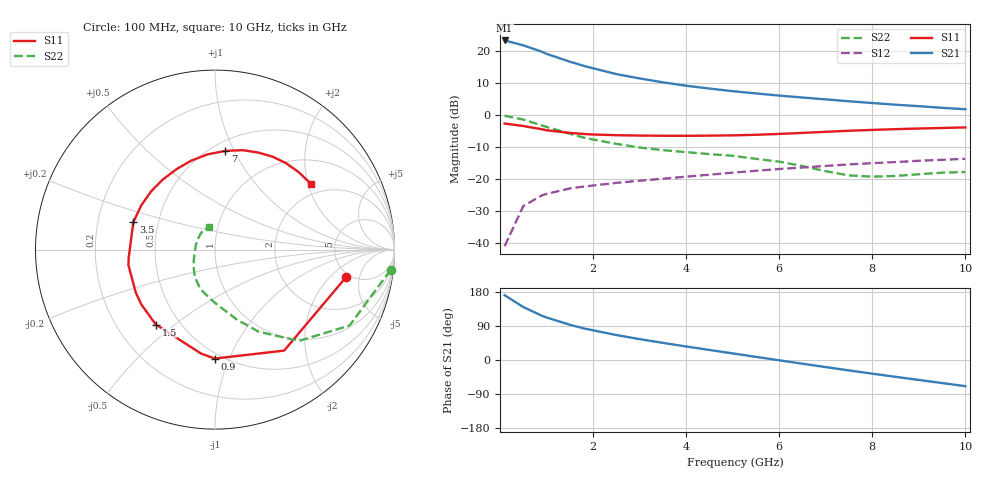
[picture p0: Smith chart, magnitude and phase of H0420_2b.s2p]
!HBFP-0420
!S-PARAMETERS at Vce=2V  Ic=5mA.  LAST UPDATED 05-29-98
# ghz s ma r 50
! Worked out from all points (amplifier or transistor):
!   23 points, 100 MHz to 10 GHz, reference 50 ohm
!   highest |S21| = 23.4 dB at 100 MHz (marker M1)
!   |S21| within 3 dB of that: start of sweep to 796.8 MHz
!   unconditionally stable (mu >= 1): 3.008 GHz to end of sweep
!   at 1 GHz: K = 0.39, MSG = 21.9 dB, |S12| = -24.6 dB
!   at 4.5 GHz: K = 1.20, MAG = 10.8 dB, |S12| = -18.6 dB
!   at 10 GHz: K = 1.24, MAG = 4.8 dB, |S12| = -13.6 dB
!   lowest NFmin = 1.00 dB at 900 MHz
!   S11 on the Smith chart (normalised r, x): 100 MHz: 4.59, -3.19; 900 MHz: 0.46, -0.89; 1.5 GHz: 0.37, -0.43; 3.5 GHz: 0.36, +0.14; 7 GHz: 0.58, +0.92; 10 GHz: 1.65, +2.09
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0.1  0.746 -11.9  14.85 171.0  0.009 84.8  0.985 -6.6
0.5  0.682 -55.6  12.47 139.8  0.038 63.6  0.861 -29.4
0.9  0.607 -90.1  9.909 116.8  0.056 49.3  0.696 -46.6
1  0.585 -97.5  9.181 112.2  0.059 46.9  0.661 -49.3
1.5  0.532 -128.3  6.918 93.1  0.072 37.2  0.516 -62.2
1.8  0.512 -143.1  5.952 83.4  0.077 33.2  0.45 -67.7
2  0.502 -151.6  5.453 78.4  0.08 31.2  0.419 -71.6
2.5  0.49 -169.8  4.422 65.8  0.088 26.9  0.359 -78.4
3  0.483 -174.6  3.786 55.2  0.095 23.4  0.314 -86.3
3.5  0.48 161.4  3.286 45.2  0.102 19.8  0.286 -92.5
4  0.479 149.2  2.908 35.7  0.11 16.3  0.266 -98.1
4.5  0.482 137.6  2.629 26.5  0.118 12.5  0.248 -104.1
5  0.487 126.5  2.389 17.4  0.127 8.1  0.233 -110.5
5.5  0.497 115.4  2.205 8.3  0.136 3.5  0.209 -117.9
6  0.513 105.0  2.04 -0.8  0.145 -1.5  0.189 -126.4
6.5  0.532 94.6  1.902 -9.8  0.153 -7.1  0.161 -137.1
7  0.553 84.0  1.778 -18.7  0.162 -12.6  0.134 -152.0
7.5  0.575 74.5  1.662 -27.5  0.171 -18.2  0.115 -171.2
8  0.592 66.0  1.559 -36.1  0.179 -24.0  0.11 167.1
8.5  0.609 58.2  1.469 -44.4  0.186 -29.8  0.113 147.2
9  0.623 50.7  1.393 -52.6  0.195 -35.4  0.12 130.6
10  0.648 34.5  1.248 -69.1  0.209 -48.0  0.13 103.9
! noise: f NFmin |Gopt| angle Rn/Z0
0.9  1  0.281  28.8  0.19
1.5  1.1  0.187  68.3  0.15
2  1.18  0.154  118.4  0.12
3  1.32  0.226  165.9  0.1
4  1.49  0.292  -162.3  0.1
5.5  1.75  0.375  -121  0.19
6.5  1.94  0.453  -98.1  0.32
7.5  2.15  0.506  -74.8  0.54
8.5  2.47  0.556  -56.8  0.83
10  2.74  0.624  -31  1.37
